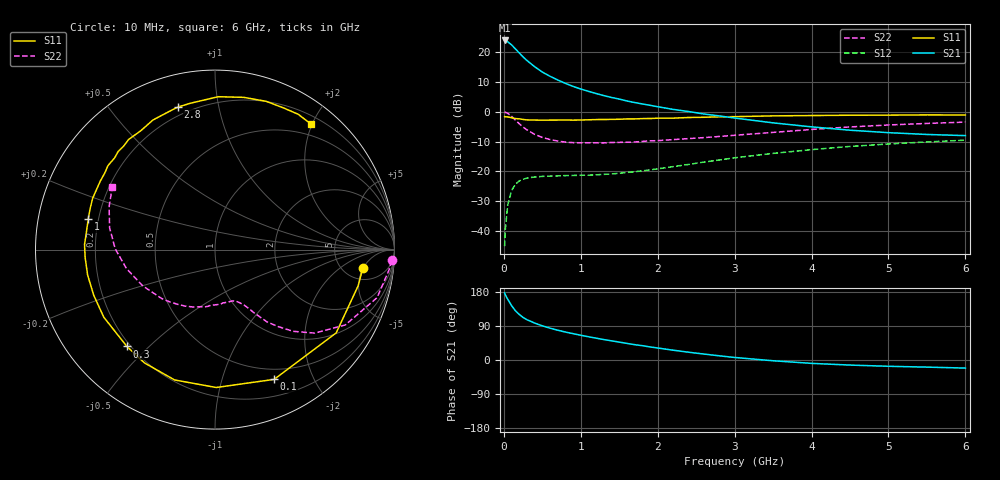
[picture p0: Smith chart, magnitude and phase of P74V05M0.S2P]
! SIEMENS Small Signal Semiconductors
! BFP196
! Si NPN RF Bipolar Junction Transistor in SOT143
! VCE = 4 V  IC = 5 mA
! Common Emitter S-Parameters:  May  1996
# GHz  S  MA  R  50
!  f  S11  S21  S12  S22
! GHz  MAG  ANG  MAG  ANG  MAG  ANG  MAG  ANG
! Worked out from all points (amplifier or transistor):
!   36 points, 10 MHz to 6 GHz, reference 50 ohm
!   highest |S21| = 23.9 dB at 10 MHz (marker M1)
!   |S21| within 3 dB of that: start of sweep to 156.7 MHz
!   unconditionally stable (mu >= 1): 1.13 GHz to 3.159 GHz
!   at 250 MHz: K = 0.25, MSG = 20.5 dB, |S12| = -22.6 dB
!   at 1.4 GHz: K = 1.15, MAG = 10.5 dB, |S12| = -20.8 dB
!   at 6 GHz: K = 1.00, MSG = 0.8 dB, |S12| = -9.5 dB
!   S11 on the Smith chart (normalised r, x): 10 MHz: 7.41, -4.95; 100 MHz: 0.38, -1.49; 300 MHz: 0.19, -0.43; 1 GHz: 0.16, +0.12; 2.8 GHz: 0.16, +0.76; 6 GHz: 0.32, +1.99
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0.01  0.83 -7.2  15.62 177.0  0.0056 86.9  0.9869 -3.5
0.02  0.8227 -14.2  15.36 171.8  0.011 81.8  0.9761 -6.7
0.05  0.8193 -34.5  14.85 160.4  0.0272 72.3  0.942 -16.5
0.1  0.7946 -65.5  13.2 143.8  0.0477 58.1  0.839 -30.0
0.15  0.7683 -89.5  11.29 129.9  0.0609 46.7  0.7251 -39.9
0.2  0.7603 -107.2  9.667 120.3  0.0692 39.5  0.6297 -46.3
0.25  0.7437 -121.9  8.264 112.3  0.0739 33.7  0.5537 -50.7
0.3  0.7294 -132.3  7.217 106.3  0.0774 30.5  0.4975 -54.2
0.4  0.7251 -148.7  5.681 97.5  0.0807 25.5  0.4176 -58.1
0.5  0.722 -159.4  4.622 90.2  0.0826 22.8  0.3713 -60.6
0.6  0.7237 -168.7  3.925 84.0  0.0835 22.1  0.3421 -63.0
0.7  0.7248 -176.5  3.405 78.6  0.0841 21.4  0.3231 -65.6
0.8  0.7274 177.8  2.986 73.8  0.0852 21.6  0.3099 -67.9
1  0.7266 166.4  2.401 65.3  0.0863 23.0  0.3014 -72.7
1.1  0.732 162.0  2.195 61.4  0.0865 24.3  0.3009 -75.6
1.6  0.7578 141.9  1.513 43.8  0.0962 32.1  0.3087 -91.2
2.2  0.7807 122.0  1.095 25.9  0.1203 39.2  0.3412 -110.2
2.8  0.8207 104.6  0.851 11.1  0.1555 39.8  0.3851 -130.7
3.5  0.852 88.8  0.651 -2.0  0.2006 34.6  0.4506 -153.4
4.5  0.8739 71.0  0.49 -13.4  0.2622 23.4  0.556 179.6
5.5  0.8851 58.4  0.416 -18.8  0.3123 10.8  0.6367 157.9
6  0.8808 52.4  0.398 -21.3  0.3338 4.1  0.67 148.6
